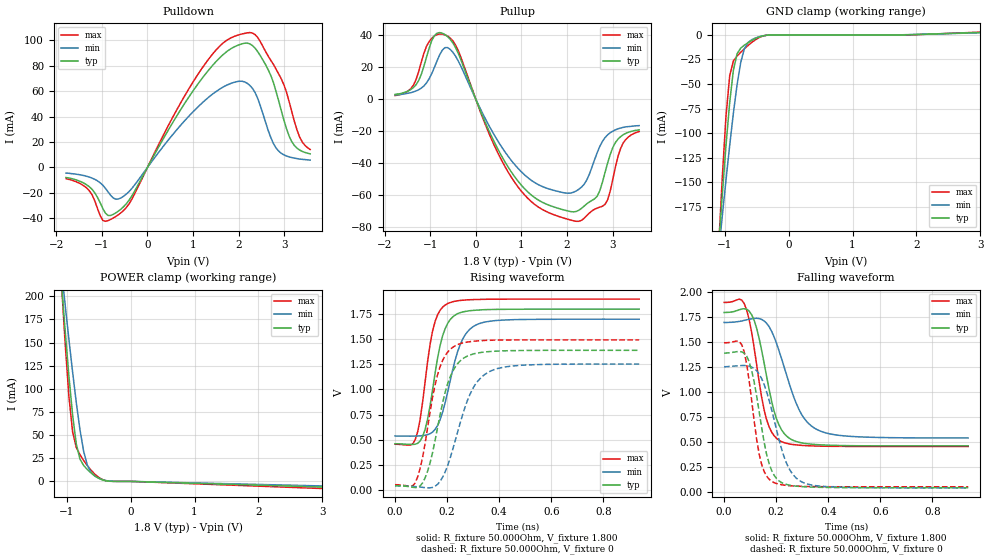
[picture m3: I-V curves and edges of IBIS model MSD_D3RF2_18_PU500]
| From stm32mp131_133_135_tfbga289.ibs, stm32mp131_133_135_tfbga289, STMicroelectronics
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[Model] MSD_D3RF2_18_PU500
Model_type   I/O
C_comp 2.391pF   2.309pF   2.512pF
Vinh = 1.150V
Vinl = 650.000mV
Vmeas = 900.000mV
Vref = 900.000mV
[Model Spec]
Vinh   1.150V   1.100V   1.200V
Vinl   650.000mV   600.000mV   700.000mV
Vmeas   900.000mV   850.000mV   950.000mV
Vref   900.000mV   850.000mV   950.000mV
[Temperature Range]   25.000   125.000   -40.000
[Voltage Range]   1.800V   1.700V   1.900V
[GND Clamp Reference]   0.00V   0.00V   0.00V
[Pulldown Reference]   0.00V   0.00V   0.00V
[POWER Clamp Reference]   1.800V   1.700V   1.900V
[Pullup Reference]   1.800V   1.700V   1.900V
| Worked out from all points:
|   slope of the pulldown table from 0 to 0.27 V, typ, clamps not added: 15.3 ohm
|   slope of the pullup table from 0 to 0.27 V, typ, clamps not added: 14.6 ohm
|   GND clamp passes 1 mA (typ) near -0.40 V on its own axis
|   POWER clamp passes 1 mA (typ) near -0.41 V on its own axis
|   rising waveform, R_fixture 50.000Ohm, V_fixture 1.800: 20-80 % time 55.9ps typ, 71.7ps min, 48.4ps max; typ from 0.459 V to 1.8 V
|   rising waveform, R_fixture 50.000Ohm, V_fixture 0: 20-80 % time 72.2ps typ, 91.8ps min, 63.4ps max; typ from 0.042 V to 1.39 V
|   falling waveform, R_fixture 50.000Ohm, V_fixture 1.800: 20-80 % time 66.6ps typ, 94.4ps min, 56.4ps max; typ from 1.8 V to 0.461 V
|   falling waveform, R_fixture 50.000Ohm, V_fixture 0: 20-80 % time 56.1ps typ, 78.2ps min, 47.2ps max; typ from 1.39 V to 0.041 V
[GND Clamp]
-1.785V   -902.2mA   -689.6mA   -1.211A
-1.094V   -215.1mA   -221.3mA   -215.9mA
-1.036V   -162.2mA   -184mA     -143.9mA
-978.8mV  -112.6mA   -147.6mA   -82.55mA
-921.2mV  -68.85mA   -112.6mA   -41.42mA
-863.6mV  -36.04mA   -79.87mA   -26.57mA
-806.1mV  -19.26mA   -50.83mA   -21.61mA
-748.5mV  -13.45mA   -27.99mA   -17.76mA
-690.9mV  -10.4mA    -13.95mA   -14.13mA
-575.8mV  -5.644mA   -4.836mA   -7.63mA
-287.9mV  -71.99uA   -121uA     -59.99uA
3.57V     3.622mA    3.119mA    4.327mA
[Power Clamp]
-1.77V    883.7mA    690.8mA    1.16A
-1.079V   212.9mA    226.9mA    212.8mA
-1.021V   161.4mA    189.7mA    147.3mA
-963.6mV  113.3mA    153.2mA    91.44mA
-906.1mV  71.54mA    118.1mA    53.38mA
-848.5mV  40.35mA    85.05mA    36.59mA
-790.9mV  24.07mA    55.67mA    28.84mA
-733.3mV  17.21mA    32.43mA    22.61mA
-618.2mV  9.105mA    9.871mA    12.13mA
-503mV    3.496mA    3.593mA    4.55mA
-330.3mV  166.1uA    345.1uA    193.6uA
3.585V    -7.27mA    -5.895mA   -9.227mA
[Pulldown]
-1.785V   -7.9mA     -4.4mA     -8.7mA
-1.267V   -15.3mA    -7.6mA     -18.6mA
-978.8mV  -32.1mA    -13.9mA    -41.44mA
-575.8mV  -32.49mA   -23.76mA   -35.41mA
1.267V    73.04mA    52.77mA    81.35mA
1.727V    90.57mA    64.38mA    99.51mA
2.245V    97.01mA    64.45mA    105.9mA
2.591V    80.71mA    35.6mA     91.02mA
2.821V    59.7mA     15.3mA     77.2mA
3.167V    20.2mA     7.8mA      43.7mA
3.339V    13.7mA     6.6mA      23.9mA
3.57V     10.7mA     5.8mA      14.1mA
[Pullup]
-1.77V    2.9mA      2.547mA    2.253mA
-1.367V   7.2mA      4.468mA    8.716mA
-1.136V   20.6mA     8.232mA    28.74mA
-906.1mV  39.61mA    19.85mA    39.39mA
-618.2mV  38.98mA    32.14mA    39.33mA
878.8mV   -49.38mA   -41.65mA   -52.88mA
1.455V    -64.25mA   -54.45mA   -68.74mA
2.203V    -70.07mA   -57.29mA   -76.21mA
2.664V    -60.55mA   -33.36mA   -67.94mA
2.836V    -45.7mA    -23.98mA   -65.64mA
3.182V    -23.3mA    -18.01mA   -30.43mA
3.585V    -19.2mA    -16.53mA   -20.22mA
[Ramp]
R_load=50.000Ohm
dV/dt_r   806.409mV/65.000ps  712.245mV/82.500ps  866.694mV/56.500ps
dV/dt_f   806.409mV/61.500ps  712.245mV/87.000ps  866.694mV/52.500ps
[Rising waveform]
R_fixture=50.000Ohm
V_fixture=1.800
V_fixture_min=1.700
V_fixture_max=1.900
0s        459.4mV    536.7mV    454.5mV
68ps      452.4mV    535.4mV    458.6mV
87ps      463.8mV    536.7mV    579.3mV
106ps     532mV      540.4mV    875.8mV
144ps     994.2mV    575.6mV    1.581V
173ps     1.437V     699.1mV    1.789V
202ps     1.658V     972.2mV    1.856V
250ps     1.765V     1.446V     1.887V
317ps     1.791V     1.65V      1.897V
938ps     1.8V       1.7V       1.9V
[Rising waveform]
R_fixture=50.000Ohm
V_fixture=0
0s        42.22mV    40.47mV    51.39mV
68ps      25.78mV    34.7mV     40.24mV
106ps     70.45mV    25mV       325.5mV
135ps     273.1mV    20.17mV    784mV
163ps     615.6mV    54.52mV    1.144V
192ps     967mV      176mV      1.335V
230ps     1.22V      479.3mV    1.434V
298ps     1.352V     1.005V     1.48V
374ps     1.38V      1.191V     1.491V
938ps     1.39V      1.253V     1.494V
[Falling waveform]
R_fixture=50.000Ohm
V_fixture=1.800
V_fixture_min=1.700
V_fixture_max=1.900
0s        1.798V     1.698V     1.899V
68ps      1.833V     1.713V     1.922V
87ps      1.831V     1.725V     1.821V
106ps     1.775V     1.735V     1.597V
135ps     1.535V     1.737V     1.1V
163ps     1.163V     1.691V     727.2mV
211ps     670.7mV    1.415V     517.4mV
288ps     496.6mV    824.2mV    467.8mV
365ps     472.2mV    614.6mV    458.3mV
938ps     460.7mV    539.7mV    454.9mV
[Falling waveform]
R_fixture=50.000Ohm
V_fixture=0
0s        1.39V      1.254V     1.494V
68ps      1.403V     1.266V     1.475V
96ps      1.307V     1.261V     1.121V
115ps     1.109V     1.238V     723.6mV
135ps     800.4mV    1.18V      376.1mV
163ps     380.9mV    1.007V     158.5mV
183ps     212.4mV    819.9mV    105.3mV
240ps     73.75mV    286.4mV    64.29mV
307ps     51.06mV    89.72mV    54.29mV
938ps     41.38mV    39.78mV    50.52mV
